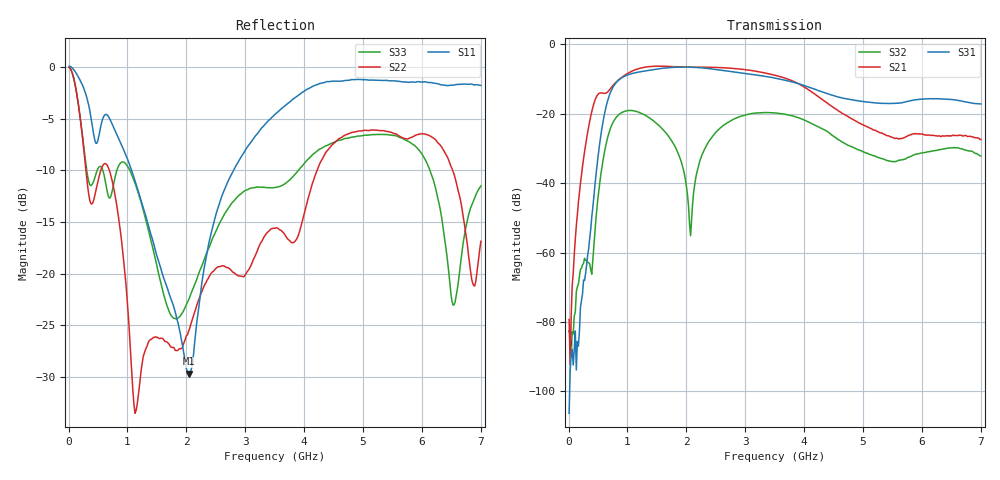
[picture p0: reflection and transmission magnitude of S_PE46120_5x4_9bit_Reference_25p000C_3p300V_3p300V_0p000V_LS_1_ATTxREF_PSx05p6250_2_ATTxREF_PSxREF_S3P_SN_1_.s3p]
! Device ID: PE46120_5x4_9bit_Reference
! Device ID: PE46120_5x4_9bit_Reference
! File Path: z:\PE46120_5x4_9bit_Reference\MPAC_Yi\new_12port\25p000C\3p300\LS_1_ATTxREF_PSx05p6250_2_ATTxREF_PSxREF\PE46120_5x4_9bit_Reference_25p000C_3p300V_3p300V_0p000V_LS_1_ATTxREF_PSx05p6250_2_ATTxREF_PSxREF_S3P_SN_1_.s3p
! Serial: 1
! Lot:
! Temp: 25.000C
! VDD: 3.300
! VSS: 0.000
! Control_Hi: 3.300
! Control_Lo: 0.000
! Logic State: LS_1_ATTxREF_PSx05p6250_2_ATTxREF_PSxREF
! Port 1: RFin
! Port 2: RFout1
! Port 3: RFout2
! ThroughPath:1-2
! IDD: -0.0005405523
! ISS: 0
! Comment:
#  Hz  S  RI  R  50
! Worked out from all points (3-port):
!   401 points, 10 MHz to 7 GHz, reference 50 ohm
!   strongest paths, dB at 10 MHz, 1.758 GHz, 3.505 GHz, 5.253 GHz, 7 GHz:
!     S31: -106.3, -6.6, -9.7, -16.9, -17.2
!     S21: -79.2, -6.4, -8.9, -25.1, -27.4
!     S32: -82.5, -28.0, -19.7, -32.5, -32.2
!   lowest |S11| = -29.7 dB at 2.037 GHz (marker M1), VSWR 1.07, Z = 52.1 + j2.58 ohm
!   |S11| at or under -10 dB: 1.069 GHz to 2.802 GHz (1.733 GHz wide, 89.5 % of centre)
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1e7  1.001 -0.1147  0.000162 1.91e-05  8.97e-05 8.57e-05
     0.000106 2.53e-05  0.989 -0.0958  -0.000116 3.92e-05
     -4.36e-06 2.12e-06  -7.4e-05 -1.13e-05  0.988 -0.0962
2.37175e8  -0.4754 -0.6621  -0.0159 -0.00624  7.29e-05 0.000204
           -0.0162 -0.00649  -0.2892 -0.3516  -0.000257 0.000648
           8.71e-05 0.000237  -0.000314 0.000588  -0.3005 -0.3522
4.6435e8  -0.4192 -0.0814  -0.0527 0.1586  0.0119 0.00396
          -0.0527 0.161  0.169 0.1868  -0.00221 0.00202
          0.0121 0.00392  -0.00218 0.00204  0.1554 0.2599
6.7405e8  -0.5626 0.1285  0.1593 0.1336  -0.0654 -0.1497
          0.1616 0.1353  0.1764 -0.2747  0.0302 -0.0379
          -0.0663 -0.1513  0.0303 -0.0384  0.2196 -0.09
1.006075e9  -0.2233 0.2757  0.3154 -0.2082  0.0106 0.3596
            0.3198 -0.2117  -0.0631 -0.0259  0.0152 0.1087
            0.0113 0.3639  0.0157 0.11  0.02 -0.3285
1.7575e9  -0.032 0.0656  -0.4721 0.0331  0.0291 -0.4598
          -0.4785 0.0336  -0.0437 -0.00309  -0.0357 0.0167
          0.0296 -0.4655  -0.0363 0.017  -0.0618 0.00155
2.0371e9  0.0214 0.0248  -0.3008 0.3553  -0.3396 -0.3189
          -0.3037 0.3605  -0.00714 0.052  0.00253 0.00376
          -0.344 -0.3221  0.00265 0.00382  -0.0741 0.00825
2.49145e9  0.0557 -0.1798  0.2469 0.3879  -0.371 0.2194
           0.2507 0.3928  0.1052 0.0019  -0.0434 0.0292
           -0.3751 0.2228  -0.044 0.0296  -0.0712 0.1409
3.505e9  -0.4517 -0.3786  -0.1181 -0.3341  0.3187 0.0541
         -0.1199 -0.3385  0.0233 0.1641  0.00275 -0.1017
         0.3227 0.0543  0.00254 -0.103  0.1867 -0.1819
7e9  -0.1164 0.8046  -0.0283 -0.0318  0.124 0.0567
     -0.0284 -0.0317  -0.0969 0.1053  0.0235 0.00578
     0.1265 0.0569  0.0239 0.00582  0.1461 0.2219
